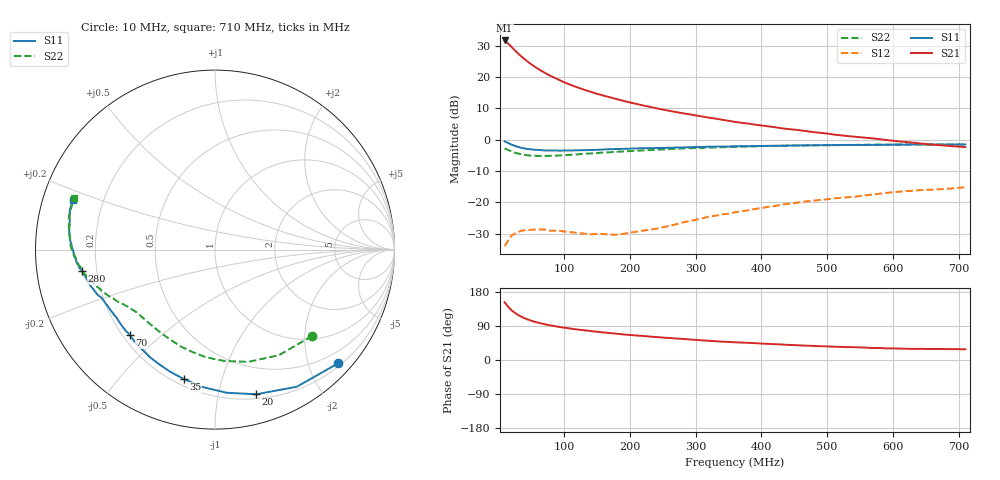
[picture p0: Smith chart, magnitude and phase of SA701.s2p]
!  POLYFET RF DEVICES
!  S PARAMETERS FOR
!  SA701
!  VDS=28, IDQ=200MA
! Date: Thu May 11 10:14:10 2000
# MHZ  S  MA  R  50.0000
! SCATTERING PARAMETERS :
! Freq=MHz Mag[s11] Ang[s11] Mag[s21] Ang[s21] Mag[s12] Ang[s12] Mag[s22] Ang[s22]
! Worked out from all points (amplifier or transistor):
!   81 points, 10 MHz to 710 MHz, reference 50 ohm
!   highest |S21| = 31.7 dB at 10 MHz (marker M1)
!   |S21| within 3 dB of that: start of sweep to 24.83 MHz
!   unconditionally stable (mu >= 1): 178 MHz to 319.2 MHz
!   at 75 MHz: K = 0.34, MSG = 24.9 dB, |S12| = -28.9 dB
!   at 310 MHz: K = 1.03, MAG = 15.2 dB, |S12| = -25.1 dB
!   at 710 MHz: K = 0.98, MSG = 6.4 dB, |S12| = -15.2 dB
!   S11 on the Smith chart (normalised r, x): 10 MHz: 0.25, -2.54; 20 MHz: 0.24, -1.30; 35 MHz: 0.24, -0.76; 70 MHz: 0.23, -0.40; 280 MHz: 0.14, -0.08; 710 MHz: 0.09, +0.17
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10  0.9345 -42.6  38.3 152.4  0.01992 63.5  0.7248 -41.5
15  0.8898 -59.2  34.39 141.3  0.02425 55.3  0.6878 -58.8
20  0.8382 -74.1  30.52 132.1  0.02923 46.9  0.6524 -73.5
25  0.7999 -85.5  27 125.1  0.03145 41.4  0.623 -85.1
30  0.7679 -95.5  24.02 119.3  0.03355 36.3  0.602 -94.7
35  0.7413 -103.7  21.45 114.6  0.03498 32.2  0.584 -102.5
40  0.7241 -110.5  19.41 110.5  0.03568 29.7  0.5733 -109.0
45  0.7095 -116.5  17.6 107.0  0.03616 26.9  0.5623 -114.6
50  0.7006 -121.1  16.09 103.9  0.03635 25.8  0.5565 -119.1
60  0.6862 -128.9  13.7 98.9  0.03655 23.0  0.5509 -126.6
70  0.6723 -135.0  11.83 94.7  0.03677 21.9  0.5515 -132.0
80  0.6712 -139.7  10.39 91.2  0.03502 22.5  0.553 -136.3
100  0.6691 -146.8  8.282 85.4  0.03419 21.6  0.5635 -142.5
130  0.679 -153.7  6.312 78.6  0.03159 26.7  0.592 -148.8
150  0.6865 -157.0  5.407 74.7  0.03134 33.5  0.6132 -151.6
180  0.7085 -160.7  4.438 69.4  0.03032 45.4  0.6391 -155.4
250  0.737 -168.1  3.022 59.2  0.03996 68.9  0.6988 -164.0
280  0.7508 -170.9  2.646 55.7  0.04754 76.3  0.7223 -166.9
360  0.7837 -177.0  1.92 46.6  0.06944 82.5  0.7688 -174.6
480  0.8114 174.9  1.315 37.1  0.1064 82.9  0.8091 175.7
600  0.8322 167.4  0.9613 30.6  0.1448 80.8  0.832 167.0
710  0.8397 160.9  0.759 28.2  0.1733 78.9  0.839 159.9
